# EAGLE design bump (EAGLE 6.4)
AUTHOR: Brad Campbell; REV: A; TITLE: Buzz
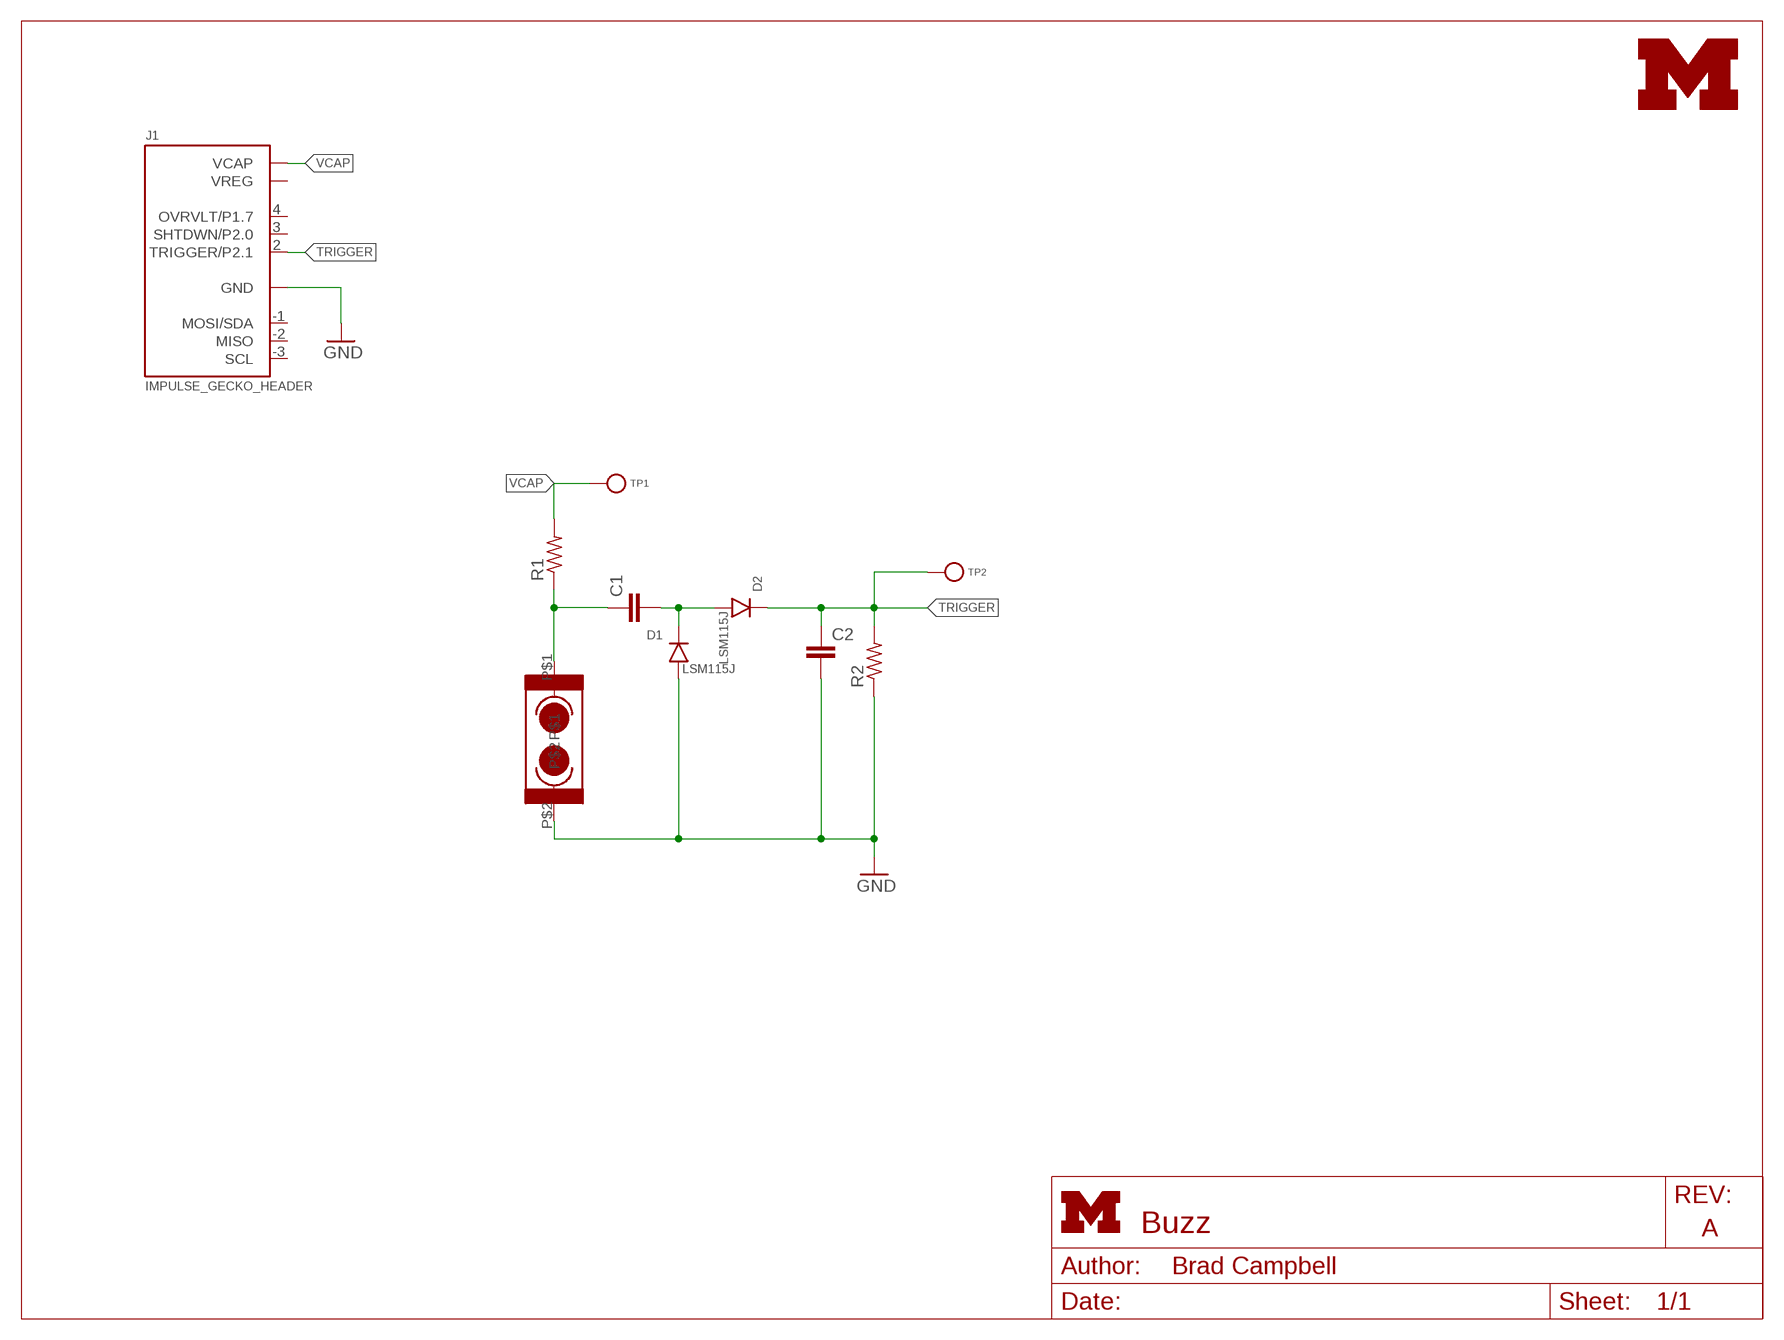
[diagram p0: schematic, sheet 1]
FRAME1 (LETTER_L): HEIGHT: 8.5in; WIDTH: 11in

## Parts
C1  C-EUC0603  [C0603]
C2  C-EUC0603  [C0603]
D1  LSM115J  [D0-214BA]
D2  LSM115J  [D0-214BA]
J1  IMPULSE_GECKO_HEADER  [HEADER1X9/0.05IN]
R1  R-US_R0603  [R0603]
R2  R-US_R0603  [R0603]
TP1  TEST_POINT_0.040IN  [TESTPOINT_0.040IN]
TP2  TEST_POINT_0.040IN  [TESTPOINT_0.040IN]
U$3  UMICH_SOLID_SMALL+  [UMICH_SOLID_100MIL]
VS1  SQ-SEN-200  [SQ-SEN-200]

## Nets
GND: C2.2 D1.A J1.0(GND) R2.1 VS1.P$2
N$1: C1.1 R1.1 VS1.P$1
N$4: C1.2 D1.C D2.A
TRIGGER: C2.1 D2.C J1.2(TRIGGER/P2.1) R2.2 TP2.TESTPOINT
VCAP: J1.5(VCAP) R1.2 TP1.TESTPOINT
Unconnected: J1.1(VREG) J1.3(SHTDWN/P2.0) J1.4(OVRVLT/P1.7) J1.-1(MOSI/SDA) J1.-2(MISO) J1.-3(SCL)

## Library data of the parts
C1 C2 = resistor:C-EU: CAPACITOR, European symbol
D1 D2 = activator:LSM115J: Diode Schottky 15V 1A; DIGIKEY: LSM115JE3/TR13CT-ND
J1 = gecko:IMPULSE_GECKO_HEADER: Header on the impulse EPIC-esque board.
R1 R2 = resistor:R-US_: RESISTOR, American symbol
TP1 TP2 = headers:TEST_POINT_0.040IN: 0.040in Test Point; DIGIKEY: 5001K-ND
U$3 = logos:UMICH_SOLID
VS1 = epic:SQ-SEN-200

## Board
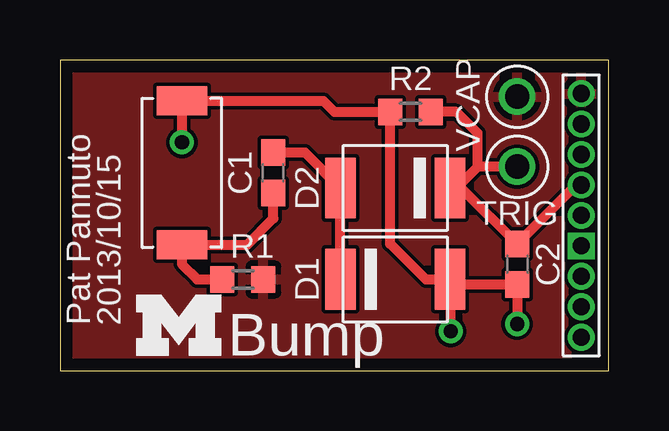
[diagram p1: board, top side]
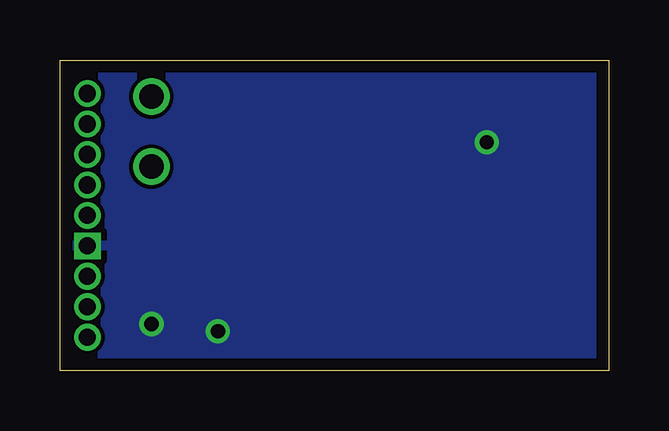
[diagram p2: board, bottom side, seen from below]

Size 22.86 x 12.95 mm. Coordinates in mm from the lower left corner, seen from the top.
Outline: 0,0 22.86,0 22.86,12.95 0,12.95 0,0
Copper layers (1*16): Top 0.0178mm / dielectric 59mil / Bottom 0.0178mm
Design rules "sunstone-2lyr_v1.0.0.3": minimum track width 6mil, minimum drill 14mil, track to track 6mil, track to pad 6mil, pad to pad 6mil, via to via 6mil, smd to smd 6mil, copper to edge 20mil, drill to drill 16mil, minimum pad ring 8mil, minimum via ring 8mil, stop-mask expansion 3mil, vias tented up to drill 0mil, thermal gap 10mil

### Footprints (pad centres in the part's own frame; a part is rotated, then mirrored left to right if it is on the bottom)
C0603 = smd 1.1 x 1: 1 -0.85,0; 2 0.85,0
D0-214BA = smd 1.27 x 2.54: A -2.286,0; C 2.286,0
HEADER1X9/0.05IN = drill 0.711 pad 1.016 square: 0 -1.27,0 | drill 0.711 pad 1.016: 1 0,0; 2 1.27,0; 3 2.54,0; 4 3.81,0; 5 5.08,0; -1 -2.54,0; -2 -3.81,0; -3 -5.08,0
R0603 = smd 1 x 1.1: 1 -0.85,0; 2 0.85,0
TESTPOINT_0.040IN = drill 1.016: TESTPOINT 0,0
SQ-SEN-200 = smd 1.2 x 2.1: P$1 -3,0; P$2 3,0

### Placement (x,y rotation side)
C1  8.89,8.26 90 top
C2  19.05,4.45 270 top
D1  13.97,3.81 180 top
D2  13.97,7.62 0 top
J1  21.72,6.48 90 top
R1  7.62,3.81 0 top
R2  14.61,10.79 0 top
TP1  19.05,11.43 0 top
TP2  19.05,8.51 0 top
U$3  3.17,0.64 0 top
VS1  5.08,8.26 90 top

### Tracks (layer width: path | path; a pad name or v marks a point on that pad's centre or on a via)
GND  (via drill 0.6)
  Top 0.406: D1.A 16.47,3.6 C2.2 v19.05,1.96 | D1.A 15.24,3.81 13.76,5.29 R2.1 11.43,10.79 10.97,11.26 VS1.P$2 v5.08,9.53 | D1.A 16.26,1.68
  other vias: 16.28,1.65
  pour Bottom: -0.64,13.97 -0.64,-1.27 23.5,-1.27 23.5,13.97
N$1
  Top 0.406: R1.1 5.71,3.81 5.08,4.45 VS1.P$1 7.79,5.25 8.89,6.35 C1.1
N$4
  Top 0.406: D1.C D2.A 10.2,9.11 C1.2
TRIGGER
  Top 0.406: J1.2 21.5,7.75 C2.1 16.73,7.62 16.51,7.62 | D2.C 16.51,7.62 | TP2.TESTPOINT 17.4,8.51 | 17.4,8.51 16.51,7.62 | 17.4,8.51 17.4,9.91 16.51,10.79 R2.2
VCAP
  pour Top: -1.27,15.24 -1.27,-2.54 24.13,-2.54 24.13,15.24

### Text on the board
tPlace: VCAP | TRIG | Pat Pannuto | 2013/10/15 | Bump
